//FC652	Send/Receive Schnittstelle - Senden
// ***************************************************************************
FUNCTION "FC_SR_SEND" : VOID

TITLE =Send/Receive Empfang

AUTHOR: 	SIEMENS
FAMILY: 	SISTARS7
VERSION: 	4.02

//KNOW_HOW_PROTECT

//Hinweis:
//Der Baustein wird vom FC651 aufgerufen. Da im FC651 der Verbindungssatz des DB984
//geladen ist darf er im FC653 nicht veraendert werden

// Datum	 Name			Aktion
// ---------------------------------------------------------------------------
// 19.05.99  Mahler		Neu



//Eingabeparameter
VAR_INPUT
	iFKT			: INT;		//Aufrufmodus
	iVBNR			: INT;		//
END_VAR

//Ausgabeparameter
//VAR_OUTPUT
//END_VAR


//Temporäre/Lokale Variable
VAR_TEMP

	anyQUEL	: ANY; 	         //Offset=0, Zeiger muss an erster Stelle stehen
	anyZIEL	: ANY;		   //Offset=10,
	uVerb		:"XC_INIT_SR_UDT";   //Offset=20
      uJob		:"XC_JOB_SR_UDT";    //Offset=70


      iLoop		: INT;
	iAct		: INT;

	bCSend	: Byte;
	bCRecv	: Byte;
	bCSave	: Byte;

      dwPTR1	: DWORD;
      dwPTR2	: DWORD;

      bTyp		: Byte;
	iDB		: INT;
	iDW		: INT;
      iAnz		: INT;

      iSendDW     : INT;
      iAnzSe	: INT;

      iJob     	: INT;
      eJob     	: INT;
      aJob		: INT;

	iDone		: INT;

      iDW1		: INT;
      iDW2		: INT;
      iDW3		: INT;
      iDW4		: INT;
      iDW5		: INT;
      iDW6		: INT;

	dwAR1		: DWORD;

END_VAR

BEGIN

NETWORK
TITLE = AR1 retten
// ===========================================================================

	TAR1	#dwAR1;

NETWORK
TITLE = Vorbesetzen der Zeiger
// ===========================================================================
//Pionter fuer den Empfangspuffer zusammenstellen
//Any-Pointer:
//Byte 0	: S7-Typ 		= 16=10H                 LB0,LB10
//Byte 1	: Datentyp		= 02=Byte			 LB1,LB11
//Byte 2/3	: Wiederholungsfaktor				 LW2,LW12
//Byte 4/5	: DB-Nummer						 LW4,LW14
//Byte 6-9	: Bereichszeiger					 LD6,LD16

	L 16;		//S7-Typ
	T LB 0;
	T LB 10;
	L 2;		//Datentyp=Byte
	T LB1;
	T LB11;


NETWORK
TITLE =Daten holen	- Verbindungsblock
// ===========================================================================

	L   #iVBNR;
	+  -1;
	L   "XC_VERB_SR".iLen;
      *I;
	L   "XC_VERB_SR".iOffset;
	+I;
	SLD 3;
	T #dwPTR1;		//Bereichszeiger

	LAR1 p#20.0;       //Pionter auf uVERB in den lokalen Daten

	auf  "XC_VERB_SR";

//Schleife um Daten in lokale Variable Byteweise umzuladen
	L  "XC_VERB_SR".iLen;		//Anzahl der Bytes
Lo21: T #iLoop;

      L DBB[#dwPTR1];		//Wert aus DB holen
	T LB [AR1,p#0.0];		//Wert in uVERB eintragen

	+AR1 p#1.0;			//AR1 um 1Bytes erhoehen
	l  #dwPTR1;			//Zeiger fuer DB-Datenwort erhoehen
	L 8;
	+D;
	T #dwPTR1;
	L   #iLoop;			//Schleifenzaehler erniedrigen und zum Anfang
	LOOP Lo21;




NETWORK
TITLE =Zyklischer Teil:  FKT 1 - Sendepuffer fuellen
// ===========================================================================

	l #iFkt;
	l 1;
	<>I;
      spb end1;
      l #uVerb.bStep;                //Nur im Schritt 0 nach Jobs suchen
      l 0;
      <>I;
      spb end1;
      L 0;
 	t #uVerb.bcount1;
 	t #uVerb.bcount2;

//*****************************
//Suchen nach Auftraegen
//*****************************

      l #uVerb.iLen;
      l 4;                    //4 Bytes Telegrammzaehler, Endekennung
      -I;
      t #iAnzSe;


a30:	l #uVerb.iPtrJobSeek;		//Letzten Pionter holen
      + 1;
     	t #uVerb.iPtrJobSeek;
	L   "XC_JOB_SR".iActSum;
      <=I;
      spb an30;
      L 1;                    	//Evtl. Grundstellung herstellen
     	t #uVerb.iPtrJobSeek;

an30: L 2;
      t #iAct;

	L 0;
      T   #eJob;

     	L #uVerb.iPtrJobSeek;
	t  #iJob;




Lo30:	L   #iJob;			//In einer Schleife nach einem Auftrag suchen
	+ -1;
      L   "XC_JOB_SR".iLen;
      *I;
	L   "XC_JOB_SR".iOffsetSys;
	+I;
	SLD 3;
	T #dwPTR1;		//Bereichszeiger
      LAR1;

	auf  "XC_JOB_SR";

	un DBX[AR1, p#3.0];		//#uJob.boEnable; Pruefen ob Block belegt dh. Zeit abgelaufen
	spb  ne32;

      L #uVerb.bPCU;            	//PCU-Nummer pruefen
      l  DBW[AR1, p#0.0];	  	//#uJob.iPCU
      <>I;
	spb ne32;

	LAR1 p#70.0;       //Pionter auf uVERB in den lokalen Daten


//Schleife um Daten in lokale Variable Byteweise umzuladen
	L  "XC_JOB_SR".iLen;		//Anzahl der Bytes
Lo31: T #iLoop;

      L DBB[#dwPTR1];		//Wert aus DB holen
	T LB [AR1,p#0.0];		//Wert in uVERB eintragen

	+AR1 p#1.0;			//AR1 um 1Bytes erhoehen
	l  #dwPTR1;			//Zeiger fuer DB-Datenwort erhoehen
	L 8;
	+D;
	T #dwPTR1;
	L   #iLoop;			//Schleifenzaehler erniedrigen und zum Anfang
	LOOP Lo31;


//****************************
// Sendepuffer eintragen
//****************************


	l #uJob.bType;		//DB senden
	l 50;
	==I;
	spb copy;
	l #uJob.bType;		//DX senden
	l 51;
	==I;
	spb copy;

	l #uJob.bType;		//DB fetch
	l 52;
	==I;
	spb fetc;
	l #uJob.bType;		//DX fetch
	l 53;
	==I;
	spb fetc;
	l #uJob.bType;		//Kettenstart
	l 54;
	==I;
	spb Kett;

	l #uJob.bType;		//Uhrzeit an S5
      l 66;
      ==I;
	spb s5DB;
	l #uJob.bType;		//Uhrzeit an S5
      l 67;
      ==I;
	spb s5DX;
	l #uJob.bType;		//Uhrzeit an S7
      l 68;
      ==I;
	spb s7DB;
      spb ne32;			//Naechsten Job pruefen

s5DB: nop 0;			//Uhrzeit an S5 DB

	L #uJob.bSrc_AREA;
	L 0;
      <>I;
      spb copy;

      L #uVerb.bPCU;          //PCU-Nummer eintragen
      t #uJob.iPCU;


      L 2;                    //Datentyp = 2Bytes
	t  #uJob.bSrc_DType;
	t  #uJob.bDest_DType;

	L B#16#84;              //Bereich = 84=DB
	t  #uJob.bSrc_AREA;
	t  #uJob.bDest_AREA;

	l  201;			//Ziel-DB
	t  #uJob.iDest_DB;
	L  701;              	//Quell-DB
	t  #uJob.iSrc_DB;

	l  182;			//Quell-DW
	t #uJob.dwSrcByte;
      l  95;			//Ziel-DW
	t #uJob.dwDestByte;

	l  8;			//Anzahl Bytes
	t #uJob.iSrc_Num;
	t #uJob.iDest_Num;

      spa copy;

s5DX: nop 0;			//Uhrzeit an S5 DB

	L #uJob.bSrc_AREA;
	L 0;
      <>I;
      spb copy;

      L #uVerb.bPCU;          //PCU-Nummer eintragen
      t #uJob.iPCU;


      L 2;                    //Datentyp = 2Bytes
	t  #uJob.bSrc_DType;
	t  #uJob.bDest_DType;

	L B#16#84;              //Bereich = 84=DB
	t  #uJob.bSrc_AREA;
	t  #uJob.bDest_AREA;

	L  701;              	//Quell-DB
	t  #uJob.iSrc_DB;

	l  182;			//Quell-DW
	t #uJob.dwSrcByte;

	l  8;			//Anzahl Bytes
	t #uJob.iSrc_Num;
	t #uJob.iDest_Num;

      spa copy;

s7DB: nop 0;			//Uhrzeit an S5 DB

	L #uJob.bSrc_AREA;
	L 0;
      <>I;
      spb copy;

      L #uVerb.bPCU;          //PCU-Nummer eintragen
      t #uJob.iPCU;


      L 2;                    //Datentyp = 2Bytes
	t  #uJob.bSrc_DType;
	t  #uJob.bDest_DType;

	L B#16#84;              //Bereich = 84=DB
	t  #uJob.bSrc_AREA;
	t  #uJob.bDest_AREA;

	L  701;              	//Quell-DB
	t  #uJob.iSrc_DB;
	t  #uJob.iDest_DB;

	l  182;			//Quell-DW
	t #uJob.dwSrcByte;
      l  190;			//Ziel-DW
	t #uJob.dwDestByte;

	l  8;			//Anzahl Bytes
	t #uJob.iSrc_Num;
	t #uJob.iDest_Num;

      spa copy;

fetc: nop 0;

      l #iAnzSe;                  //Auftrag geht nicht in den Sendepuffer
      l 8;				    // - 8 Bytes Header
      -I;
	l 12;				    // - Anzahl Bytes Nutzdaten = Fetchauftrag mit 12 Bytes
      -I;				    //  Ein Fetch-Auftrag besteht aus dem Header mit 8 Bytes
      l 0;                        //  und 12 Bytes Nutzdaten in denen der Job eingetragen wird
      <I;
      spb end1;

	l #uVerb.iSendDW;
      l #iAct;
	+I;
	sld 3;
      T   #dwPTR1;

	auf DB[#uVerb.iSendDB];

	l #uJob.bType;			//AuftragZiel - Header im Sendepuffer
      t  DBB[#dwPTR1];

	l #dwPTR1;
	l 8;
	+d;
	t #dwPTR1;

	l #uJob.bType;		//AuftragQuelle - Header im Sendepuffer
      t  DBB[#dwPTR1];


	l #dwPTR1;
	l 8;
	+d;
	t #dwPTR1;

	l  #uJob.iDest_DB;	//Ziel DB - Header im Sendepuffer
      t  DBW[#dwPTR1];

	l #dwPTR1;
	l 16;
	+d;
	t #dwPTR1;

	l  #uJob.dwDestByte; 	//Ziel DW - Header im Sendepuffer
      t  DBW[#dwPTR1];

	l #dwPTR1;
	l 16;
	+d;
	t #dwPTR1;

	L 6;
      t  DBW[#dwPTR1];        //Anzahl Datenworte = 6  - Header im Sendepuffer

 	l #dwPTR1;
	l 16;
	+d;
	t #dwPTR1;

	l #uJob.bType;				//AuftragZiel - Nutzdaten 1 im Sendepuffer
      t  DBB[#dwPTR1];

	l #dwPTR1;
	l 8;
	+d;
	t #dwPTR1;

	l #uJob.bType;		//AuftragQuelle - Nutzdaten 1 im Sendepuffer
      t  DBB[#dwPTR1];

	l #dwPTR1;
	l  8;
	+d;
	t #dwPTR1;

	l  #uJob.iDest_DB;	//Ziel DB - Nutzdaten 2 im Sendepuffer
      t  DBW[#dwPTR1];

	l #dwPTR1;
	l 16;
	+d;
	t #dwPTR1;

	l  #uJob.dwDestByte; 	//Ziel DW - Nutzdaten 3 im Sendepuffer
      t  DBW[#dwPTR1];

	l #dwPTR1;
	l 16;
	+d;
	t #dwPTR1;


	l #uJob.iSrc_Num;		//Anzahl Bytes - Nutzdaten 4 im Sendepuffer
      srw 1;
      t  DBW[#dwPTR1];        //Anzahl Datenworte

	l #dwPTR1;
	l 16;
	+d;
	t #dwPTR1;


	l  #uJob.iSrc_DB;		//Quelle DB - Nutzdaten 5 im Sendepuffer
      t  DBW[#dwPTR1];

	l #dwPTR1;
	l 16;
	+d;
	t #dwPTR1;

	l #uJob.dwSrcByte;	//Quelle DW  - Nutzdaten 6 im Sendepuffer
	t  DBW[#dwPTR1];


      l 12;
	t #iAnz;

	s #uVerb.boQuitt;             //Ein Fetch-Auftrag ist fertig, wenn Partner mindestens
						//ein Anworttelegramm gesendet hat.

      spa fe31;

Kett: u #uVerb.boS7;
	spb KS7;
	u  #uVerb.boS5;
	spb KS5;
      spa ne31;

KS5:	l #iAnzSe;                  //Auftrag geht nicht in den Sendepuffer
      l 8;				    // - 8 Bytes Header
      -I;
	l 12;				    // - Anzahl Bytes Nutzdaten = Fetchauftrag mit 12 Bytes
      -I;				    //  Ein Auftrag besteht aus dem Header mit 8 Bytes
      l 0;                        //  und 12 Bytes Nutzdaten in denen der Job eingetragen wird
      <I;
      spb end1;

      l   #uJob.dwSrcByte;
	+ -8;
	sld 3;
	LAR1;

	l #uVerb.iSendDW;
      l #iAct;
	+I;
	sld 3;
      T   #dwPTR1;

	auf DB[#uVerb.iSendDB];
	l #uJob.bType;			//AuftragZiel - Header im Sendepuffer
      t  DBB[#dwPTR1];

	l #dwPTR1;
	l 8;
	+d;
	t #dwPTR1;

	auf DB [#uJob.iSrc_DB];
	L  DBB[AR1,p#11.0];		//Ziel-Teilanlage - Header im Sendepuffer
	auf DB[#uVerb.iSendDB];
      t  DBB[#dwPTR1];

	l #dwPTR1;
	l 8;
	+d;
	t #dwPTR1;
	L 6;
	t  DBW[#dwPTR1];			//Reserve - Header im Sendepuffer immer ungleich 0

	l #dwPTR1;
	l 16;
	+d;
	t #dwPTR1;
	L 6;
	t  DBW[#dwPTR1];			//Anzahl - Header im Sendepuffer

	l #dwPTR1;
	l 16;
	+d;
	t #dwPTR1;
	L 6;
	t  DBW[#dwPTR1];			//Anzahl - Header im Sendepuffer

	l #dwPTR1;
	l 16;
	+d;
	t #dwPTR1;
	auf DB [#uJob.iSrc_DB];
	L  DBB[AR1,p#0.0];
	auf DB[#uVerb.iSendDB];
	t  DBW[#dwPTR1];			//Starttyp

	l #dwPTR1;
	l 16;
	+d;
	t #dwPTR1;
	auf DB [#uJob.iSrc_DB];
	L  DBB[AR1,p#3.0];
	auf DB[#uVerb.iSendDB];
	t  DBW[#dwPTR1];			//Quellteilanlage

	l #dwPTR1;
	l 16;
	+d;
	t #dwPTR1;
	auf DB [#uJob.iSrc_DB];
	L  DBW[AR1,p#12.0];
	auf DB[#uVerb.iSendDB];
	t  DBW[#dwPTR1];			//Jahr/Rezeptyp

	l #dwPTR1;
	l 16;
	+d;
	t #dwPTR1;
	auf DB [#uJob.iSrc_DB];
	L  DBW[AR1,p#14.0];
	auf DB[#uVerb.iSendDB];
	t  DBW[#dwPTR1];			//Rezeptnummer

	l #dwPTR1;
	l 16;
	+d;
	t #dwPTR1;
	auf DB [#uJob.iSrc_DB];
	L  DBW[AR1,p#16.0];
	auf DB[#uVerb.iSendDB];
	t  DBW[#dwPTR1];			//Auftragsnummer

	l #dwPTR1;
	l 16;
	+d;
	t #dwPTR1;
	auf DB [#uJob.iSrc_DB];
	L  DBW[AR1,p#18.0];
	auf DB[#uVerb.iSendDB];
	t  DBW[#dwPTR1];			//Chargennummer

	l 12;
	t #iAnz;				//12-Bytes Nutzdaten

	spa fe31;

KS7:   Nop 0;

	l #iAnzSe;                  //Auftrag geht nicht in den Sendepuffer
      l 8;				    // - 8 Bytes Header
      -I;
	l 12;				    // - Anzahl Bytes Nutzdaten = Fetchauftrag mit 12 Bytes
      -I;				    //  Ein Auftrag besteht aus dem Header mit 8 Bytes
      l 0;                        //  und 12 Bytes Nutzdaten in denen der Job eingetragen wird
      <I;
      spb end1;

      l   #uJob.dwSrcByte;
	+ -8;
	sld 3;
	LAR1;

	l #uVerb.iSendDW;
      l #iAct;
	+I;
	sld 3;
      T   #dwPTR1;

	auf DB[#uVerb.iSendDB];
	l  50;			//Auftrags Art - Header im Sendepuffer
      t  DBB[#dwPTR1];		//Sende DB

	l #dwPTR1;
	l 8;
	+d;
	t #dwPTR1;

	l  50;			//Auftrags Art - Header im Sendepuffer
      t  DBB[#dwPTR1];		//Sende DB


	l #dwPTR1;
	l 8;
	+d;
	t #dwPTR1;
	L  988;
	t  DBW[#dwPTR1];		//DB-Nummer - Header im Sendepuffer

	l #dwPTR1;
	l 16;
	+d;
	t #dwPTR1;
	auf DB [#uJob.iSrc_DB];
	L  DBB[AR1,p#11.0];
	+ -1;
	l  "XC_RASTA_SR".iLen;
	*I;
	l  "XC_RASTA_SR".iOffset;
	+I;
	auf DB[#uVerb.iSendDB];
	t  DBW[#dwPTR1];			//DW-Nummer - Header im Sendepuffer

	l #dwPTR1;
	l 16;
	+d;
	t #dwPTR1;
	L 6;
	t  DBW[#dwPTR1];			//Anzahl - Header im Sendepuffer

	l #dwPTR1;
	l 16;
	+d;
	t #dwPTR1;
	auf DB [#uJob.iSrc_DB];
	L  DBW[AR1,p#8.0];
	auf DB[#uVerb.iSendDB];
	t  DBW[#dwPTR1];			//Quell-PCU-Nummer und Ziel-PCU-Nummer

	l #dwPTR1;
	l 16;
	+d;
	t #dwPTR1;
	auf DB [#uJob.iSrc_DB];
	L  DBW[AR1,p#10.0];
	auf DB[#uVerb.iSendDB];
	t  DBW[#dwPTR1];			//Quell-ASTA, Zeil-Teilanlage

	l #dwPTR1;
	l 16;
	+d;
	t #dwPTR1;
	auf DB [#uJob.iSrc_DB];
	L  DBW[AR1,p#12.0];
	auf DB[#uVerb.iSendDB];
	t  DBW[#dwPTR1];			//Jahr, Rezepttyp

	l #dwPTR1;
	l 16;
	+d;
	t #dwPTR1;
	auf DB [#uJob.iSrc_DB];
	L  DBW[AR1,p#14.0];
	auf DB[#uVerb.iSendDB];
	t  DBW[#dwPTR1];			//Rezeptnummer

	l #dwPTR1;
	l 16;
	+d;
	t #dwPTR1;
	auf DB [#uJob.iSrc_DB];
	L  DBW[AR1,p#16.0];
	auf DB[#uVerb.iSendDB];
	t  DBW[#dwPTR1];			//Auftragsnummer

	l #dwPTR1;
	l 16;
	+d;
	t #dwPTR1;
	auf DB [#uJob.iSrc_DB];
	L  DBW[AR1,p#18.0];
	auf DB[#uVerb.iSendDB];
	t  DBW[#dwPTR1];			//Chargennummer

	l 12;
	t #iAnz;				//12-Bytes Nutzdaten

	spa fe31;



copy: nop 0;

      l #iAnzSe;                  //Auftrag geht nicht in den Sendepuffer
      l 8;				    // - 8 Bytes Header
      -I;
	l #uJob.iSrc_Num;		    // - Anzahl Bytes Nutzdaten
      -I;
      l 0;
      <I;
      spb end1;

	l #uVerb.iSendDW;
      l #iAct;
	+I;
	sld 3;
      T   #dwPTR1;

	auf DB[#uVerb.iSendDB];

	l #uJob.bType;		//AuftragZiel - Header im Sendepuffer
      t  DBB[#dwPTR1];

	l #dwPTR1;
	l 8;
	+d;
	t #dwPTR1;

	l #uJob.bType;			//AuftragQuelle - Header im Sendepuffer
      t  DBB[#dwPTR1];

	l #dwPTR1;
	l 8;
	+d;
	t #dwPTR1;

	l  #uJob.iDest_DB;	//Ziel DB - Header im Sendepuffer
      t  DBW[#dwPTR1];

	l #dwPTR1;
	l 16;
	+d;
	t #dwPTR1;

	l  #uJob.dwDestByte; 	//Ziel DW - Header im Sendepuffer
      t  DBW[#dwPTR1];

	l #dwPTR1;
	l 16;
	+d;
	t #dwPTR1;

	l #uJob.iSrc_Num;		//Anzahl Bytes - Header im Sendepuffer
      srw 1;
      t  DBW[#dwPTR1];        //Anzahl Datenworte


	l #uVerb.iSendDW;		//Anfang Sendepuffer
      l #iAct;			// + Offset
	+I;
      l 8;				//Header
      +I;
      t #iSendDW;

	l  #uJob.iSrc_DB;		//Quelle DB
      t  #iDB;

	l #uJob.dwSrcByte;	//Quelle DW
	t  #iDW;

	l #uJob.iSrc_Num;		//Anzahl Bytes
      t #iAnz;


	  call "FC_COPY" (      //Nutzdaten
                      iQDB	:=#iDB,
			    iQDW	:=#iDW,
                      bQTyp   :=b#16#84,
			    iZDB	:=#uVerb.iSendDB,
		          iZDW	:=#iSendDW,
                      bZTyp   :=b#16#84,
			    iLenByte:=#iAnz
			    );

      l #iAnz;           //Pruefen ob Sendepuffer beschrieben wurde
      l 0;
      <>I;
      spb fe31;
      u #uJob.boEnable;
	r #uJob.boEnable;        //Block freigeben
      s #uJob.boParamError;

	l   #iJob;
	t    #uVerb.iPtrJob;	       //Pointer speichern der Fundstelle

      spa ne31;


fe31: l #iAct;			//Offset z.B 2
      l #iAnz;                //Anzahl in Bytes
      +I;
      l 8;				//Header 8 Bytes
      +I;
      t #iAct;			//Neuer Offset im Sendepuffer fuer Endezeichen oder neuen Auftrag

	l #iAnzSe;                  //Restlaenge des Sendepuffer
      l 8;				    // - 8 Bytes Header
      -I;
	l #iAnz;		    // - Anzahl Bytes Nutzdaten
      -I;
      t #iAnzSe;                  //Neue Restlaenge des Sendepuffer


	l #uVerb.iSendDW;       //Anfang Sendepuffer
      l #iAct;			//Offset z.B 2
      +I;
	sld 3;
	t #dwPTR1;

	l -1;
	t  DBW[#dwPTR1];        //Endekennung

//****************************
// Kennung Senden ausfuehren
//****************************

      l 1;
      t #uVerb.bStep;                //Schritt = 1 setzen



	l   #iJob;
	t    #uVerb.iPtrJob;	       //Pointer speichern der Fundstelle


      u #uJob.boEnable;
	r #uJob.boEnable;        //Block freigeben
	R #uJob.boParamError;

	L #uJob.bType;           //Bei Kettenstart oder Job mit Quittung
	L 54;                    //Kennung Quittung in die Verbindung
	==I;
      o #uJob.boQuit;
      s #uVerb.boQuitt;


      un #uJob.boTmpJob;        //Pruefen ob Block nur einmal bearbeiten
      spb ne31;
      r #uJob.boTmpJob;

      l 0;
      T  #uJob.iPCU;



//***********************
//Auftragsblock zurueck
//***********************


ne31:	L   #iJob;			//In einer Schleife Block zurueckschreiben
	+  -1;
	L   "XC_JOB_SR".iLen;
      *I;
	L   "XC_JOB_SR".iOffsetSys;
	+I;
	SLD 3;
	T #dwPTR1;		//Bereichszeiger

	LAR1 p#70.0;       //Pionter auf uJob in den lokalen Daten

	auf  "XC_JOB_SR";

	L  "XC_JOB_SR".iLen;		//Anzahl der Bytes
Lo32: T #iLoop;

  	l LB [AR1,p#0.0];		//Wert in uJob eintragen
      T DBB[#dwPTR1];		//Wert aus DB holen

	+AR1 p#1.0;			//AR1 um 1Bytes erhoehen
	l  #dwPTR1;			//Zeiger fuer DB-Datenwort erhoehen
	L 8;
	+D;
	T #dwPTR1;
	L   #iLoop;			//Schleifenzaehler erniedrigen und zum Anfang
	LOOP Lo32;


ne32: l   #iJob;			//Naechsten Systemjob anwaehlen
      T #uVerb.iPtrJobSeek;
	+ 1;
      t   #iJob;
	L   "XC_JOB_SR".iActSum;
      <=I;
      spb pr32;
      l 1;
      t  #iJob;

pr32:	L   #eJob;              //Pro Zyklus alle Auftraege bearbeiten
	+ 1;
      T   #eJob;
    	L   "XC_JOB_SR".iActSum;
      <I;
      spb Lo30;


end1: nop 0;

NETWORK
TITLE =Pruefen ob Quittung eingetragen werden muss		STEP 1
// ===========================================================================
      l #iFKT;
	L 1;
	<>I;
	spb ende;
	l #uVerb.bStep;                //Nur im Schritt 1 pruefen ob Telegrammzaehler
      l 1;                           //erhoeht werden muss
	<>I;
      spb ende;
      l 2;
	t #uVerb.bStep;

     	s #uVerb.boSEPU;			//Sendepuffer voll dh. senden starten FC151

	un #uVerb.boQuitt;
      spb ende;

      auf DB[#uVerb.iSendDB];
      l #uVerb.iSendDW;
      + 1;
	sld 3;
	T #dwPTR1;


      l DBB[#dwPTR1];    //Telegrammzaehler erhoehen
      inc 1;
      t DBB[#dwPTR1];


ende: nop 0;

NETWORK
TITLE =Warten ob Senden fertig		STEP 2
// ===========================================================================
      l #iFKT;
	L 1;
	<>I;
	spb end3;
	l #uVerb.bStep;                //Nur im Schritt 2 Senden ueberwachen
      l 2;
	<>I;
      spb end3;
      u  #uVerb.boSendDone;           //Sendung fertig ohne Fehler
      un #uVerb.boSEPU;               //Sendung laeuft noch
      spb fer3;
      u  #uVerb.boSendERROR;          //Sendung fertig mit Fehler
      spb feh3;
      spb end3;
feh3: l #uVerb.bCount2;               //Warten auf Reaktion von Sender
      + 1;
      t #uVerb.bcount2;
      s #uVerb.boERROR;
      spb end3;

fer3: l uVerb.bSendCount;		  //Telegrammzaehler erhoehen
      + 1;
 	t uVerb.bSendCount;
	L 3;					  //Schritt 3 anwaehlen dh. warten auf Quittung
	t #uVerb.bStep;
      l 0;
 	t #uVerb.bcount1;
end3: nop 0;


NETWORK
TITLE =Warten auf Quittung			STEP 3
// ===========================================================================
      l #iFKT;
	L 1;
	<>I;
	spb end4;
	l #uVerb.bStep;                //Nur im Schritt 3 auf die Quittung warten
      l 3;
	<>I;
      spb end4;
      un  #uVerb.boQuitt;            //Pruefen ob Quittung kommen muss
      spb fer4;

      auf DB[#uVerb.iSendDB];        //Telegrammzaehler der gesendet wurde
      l #uVerb.iSendDW;              //wurde steht im Sendepuffer Byte 1
	+ 1;
	sld 3;
	T #dwPTR1;

	l DBB[#dwPTR1];
      t #iDW1;

      auf DB[#uVerb.iRecvDB];        //Telegrammzaehler der empfangen wurde
      l #uVerb.iRecvDW;              //als Spiegelung des gesendeten Tel.-Zaehler
      					 //steht im Empfangspuffer Byte 0
	sld 3;
	T #dwPTR2;
	l DBB[#dwPTR2];
      t #iDW2;


      l #iDW1;                       //Empfang gleich Senden dh. beenden
      l #iDW2;
      ==I;
      spb fer4;

	l #uVerb.bcount1;			//Warten auf Quittung
      + 1;
 	t #uVerb.bcount1;
      l 5;
      <I;
      spb end4;
      l 0;
 	t #uVerb.bcount1;

	l 1;					//Sendung mit neuem Zaehler wiederholen
 	t #uVerb.bStep;

      l #uVerb.bcount2;             //Umschaltung der Schnittstelle vorbereiten
      + 1;
 	t #uVerb.bcount2;
      spa end4;

fer4: nop 0;
	L 0;					  //Schritt 0  dh. Senden fertig
	t #uVerb.bStep;
 	t #uVerb.bcount1;
 	t #uVerb.bcount2;

	r  #uVerb.boQuitt;
      r  #uVerb.boERROR;



end4: nop 0;



NETWORK
TITLE =Schnittstelle wechseln
// ===========================================================================
      l #iFKT;
	L 1;
	<>I;
	spb end5;
	l #uVerb.bCount2;               //Pruefen ob Umschaltzaehler abgelaufen
      l 5;
	<I;
      spb end5;
      l 0;
      t #uVerb.bCount2;
      s #uVerb.boERROR;

     	l #uVerb.bRPCU;                //Umschalten nur moeglich wenn Res. PCU vorhanden
      l 0;
	==I;
      spb end5;
      u #uVerb.boAAktiv;               //Pruefen ob Normale Schnittstelle aktiv ist
      spb res;
      u #uVerb.boRAktiv;               //Pruefen ob Reserve Schnittstelle aktiv ist
      spb nor;
	spb end5;
res:  l #uVerb.bRPCU;                //Umschalten nur moeglich wenn Res. PCU vorhanden
      l 0;
	==I;
      spb end5;
      u #uVerb.boRS5;
	= #uVerb.boS5;
	u #uVerb.boRS7;
	= #uVerb.boS7;
      l #uVerb.bRPCU;
      t #uVerb.bPCU;
      l #uVerb.iRID;
      t #uVerb.iID;
   	l #uVerb.wRLADDR;
      t #uVerb.wLADDR;
	u #uVerb.boAAktiv;
	r #uVerb.boAAktiv;
      s #uVerb.boRAktiv;
	spa end5;
nor:  l #uVerb.bAPCU;                //Umschalten nur moeglich wenn Res. PCU vorhanden
      l 0;
	==I;
      spb end5;
      u #uVerb.boAS5;
	= #uVerb.boS5;
	u #uVerb.boAS7;
	= #uVerb.boS7;
      l #uVerb.bAPCU;
      t #uVerb.bPCU;
      l #uVerb.iAID;
      t #uVerb.iID;
   	l #uVerb.wALADDR;
      t #uVerb.wLADDR;
	u #uVerb.boRAktiv;
	r #uVerb.boRAktiv;
      s #uVerb.boAAktiv;
end5: nop 0;

NETWORK
TITLE =Daten zureuck	- Verbindungsblock
// ===========================================================================

	L   #iVBNR;
	+  -1;
	L   "XC_VERB_SR".iLen;
      *I;
	L   "XC_VERB_SR".iOffset;
	+I;
	SLD 3;
	T #dwPTR1;		//Bereichszeiger

	LAR1 p#20.0;       //Pionter auf uVERB in den lokalen Daten

	auf  "XC_VERB_SR";

//Schleife um Daten in lokale Variable Byteweise umzuladen
	L  "XC_VERB_SR".iLen;		//Anzahl der Bytes
Lo91: T #iLoop;

	l LB [AR1,p#0.0];		//Wert in uVERB eintragen
      T DBB[#dwPTR1];		//Wert aus DB holen

	+AR1 p#1.0;			//AR1 um 1Bytes erhoehen
	l  #dwPTR1;			//Zeiger fuer DB-Datenwort erhoehen
	L 8;
	+D;
	T #dwPTR1;
	L   #iLoop;			//Schleifenzaehler erniedrigen und zum Anfang
	LOOP Lo91;


NETWORK
TITLE = AR1 zurück, ENDE
// ===========================================================================

	LAR1	#dwAR1;

END_FUNCTION
